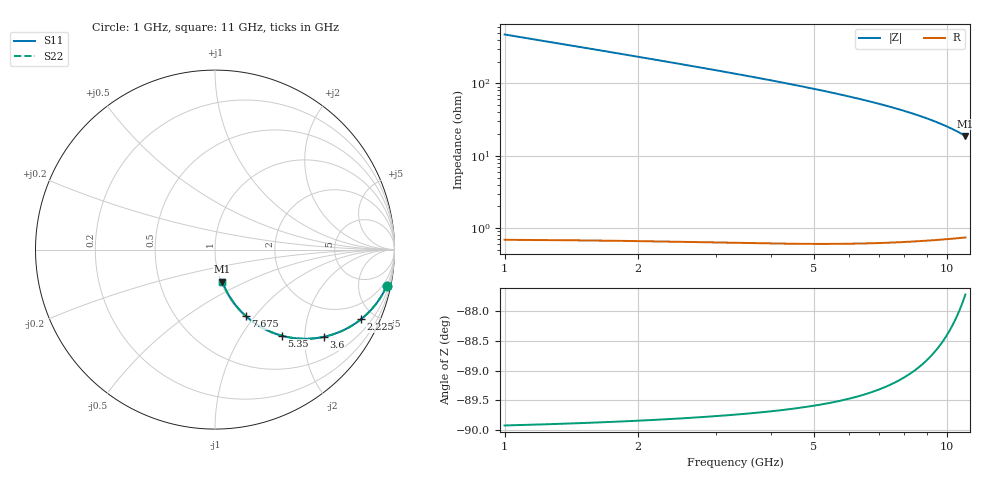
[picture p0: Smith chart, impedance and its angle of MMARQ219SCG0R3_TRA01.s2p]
! MMARQ219SCG0R3_TRA01  S-PARAMETER MODEL  ( General Type )
! Model Generated by TAIYO YUDEN Corporation (http://www.ty-top.com)
! Version 1.0
! TAIYO YUDEN Control No. 210622
! Copyright(c) 2016 TAIYO YUDEN CO.,LTD. All Rights Reserved.
! Product Description (link to TY-COMPAS)
! https://ds.yuden.co.jp/TYCOMPAS/or/detail?pn=MMARQ219SCG0R3ATRA01&u=M
! Products Name : Multilayer Ceramic Capacitors
! Characteristics :
!  Capacitance : 0.3 pF , Rated Voltage : 250V , TCC : CG / C0G
!  Case Size : 2.0 x 1.25 / 0.079 x 0.049 [mm/inch] , Thickness : 0.85 / 0.033 [mm/inch]
!  (Conditions: Temperature = 25 degC , DC Bias Current/Voltage = 0A / 0V)
! External Node Assignments :
!  1  o---| |---o  2
! GND o---------o GND
! Frequency Range : 1000MHz  -  11000MHz  [ 401 STEP ]
# MHZ S RI R 50
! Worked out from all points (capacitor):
!   401 points, 1 GHz to 11 GHz, reference 50 ohm
!   read as one part in series: C = 338 fF near 1.05 GHz
!   lowest |Z| = 18.8 ohm at 11 GHz (marker M1)
!   S11 on the Smith chart (normalised r, x): 1 GHz: 1.01, -9.47; 2.225 GHz: 1.01, -4.18; 3.6 GHz: 1.01, -2.48; 5.35 GHz: 1.01, -1.54; 7.675 GHz: 1.01, -0.90; 11 GHz: 1.01, -0.38
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1000  0.9571 -0.202  0.0429 0.202  0.0429 0.202  0.9571 -0.202
1050  0.9528 -0.2113  0.0472 0.2113  0.0472 0.2113  0.9528 -0.2113
1175  0.9415 -0.2339  0.0585 0.2339  0.0585 0.2339  0.9415 -0.2339
1300  0.9291 -0.2557  0.0709 0.2557  0.0709 0.2557  0.9291 -0.2557
1550  0.9016 -0.2968  0.0984 0.2968  0.0984 0.2968  0.9016 -0.2968
1700  0.8835 -0.3196  0.1165 0.3196  0.1165 0.3196  0.8835 -0.3196
1875  0.8611 -0.3445  0.1389 0.3445  0.1389 0.3445  0.8611 -0.3445
2225  0.8129 -0.3884  0.1871 0.3884  0.1871 0.3884  0.8129 -0.3884
2675  0.7466 -0.4331  0.2534 0.4331  0.2534 0.4331  0.7466 -0.4331
3125  0.6781 -0.465  0.3219 0.465  0.3219 0.465  0.6781 -0.465
3600  0.6063 -0.4861  0.3937 0.4861  0.3937 0.4861  0.6063 -0.4861
3975  0.5514 -0.4946  0.4486 0.4946  0.4486 0.4946  0.5514 -0.4946
4350  0.4988 -0.497  0.5012 0.497  0.5012 0.497  0.4988 -0.497
4825  0.4365 -0.4925  0.5635 0.4925  0.5635 0.4925  0.4365 -0.4925
5350  0.3737 -0.4799  0.6263 0.4799  0.6263 0.4799  0.3737 -0.4799
6000  0.305 -0.4558  0.695 0.4558  0.695 0.4558  0.305 -0.4558
6825  0.232 -0.4164  0.768 0.4164  0.768 0.4164  0.232 -0.4164
7675  0.1715 -0.3699  0.8285 0.3699  0.8285 0.3699  0.1715 -0.3699
8475  0.1264 -0.3236  0.8736 0.3236  0.8736 0.3236  0.1264 -0.3236
9350  0.0882 -0.2724  0.9118 0.2724  0.9118 0.2724  0.0882 -0.2724
10175  0.0609 -0.2249  0.9391 0.2249  0.9391 0.2249  0.0609 -0.2249
11000  0.0407 -0.1788  0.9593 0.1788  0.9593 0.1788  0.0407 -0.1788
